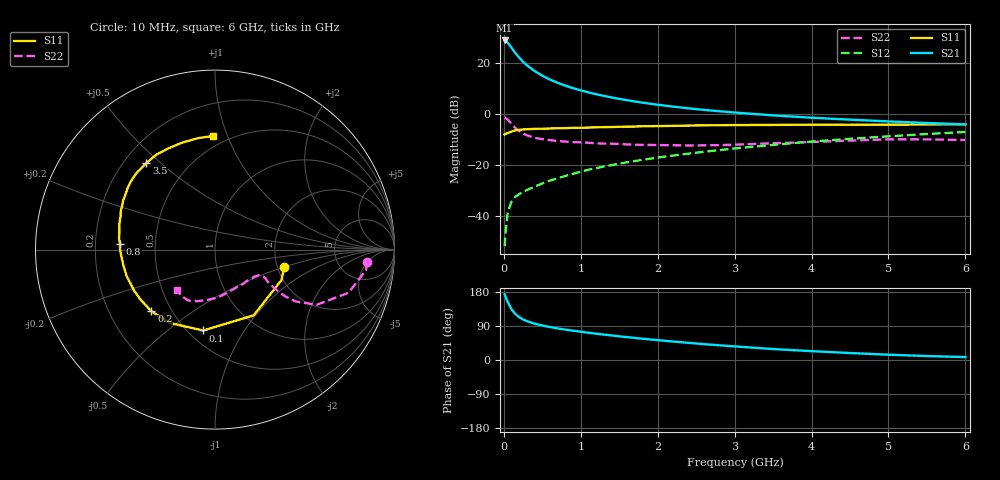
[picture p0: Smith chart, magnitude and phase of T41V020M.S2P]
! Infineon Technologies  Discrete & RF Semiconductors
! BFR182T
! Si NPN RF Bipolar Junction Transistor in SC75
! VCE = 1 V  IC = 20 mA
! Common Emitter S-Parameters:  October  1999
# GHz  S  MA  R  50
!  f  S11  S21  S12  S22
! GHz  MAG  ANG  MAG  ANG  MAG  ANG  MAG  ANG
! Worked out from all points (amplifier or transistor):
!   36 points, 10 MHz to 6 GHz, reference 50 ohm
!   highest |S21| = 29.1 dB at 10 MHz (marker M1)
!   |S21| within 3 dB of that: start of sweep to 102.8 MHz
!   unconditionally stable (mu >= 1): start of sweep to 18.1 MHz; 280.5 MHz to end of sweep
!   at 250 MHz: K = 0.94, MSG = 25.7 dB, |S12| = -30.7 dB
!   at 1.4 GHz: K = 1.48, MAG = 9.3 dB, |S12| = -20.1 dB
!   at 6 GHz: K = 1.11, MAG = -0.5 dB, |S12| = -7.0 dB
!   S11 on the Smith chart (normalised r, x): 10 MHz: 2.18, -0.50; 100 MHz: 0.59, -0.67; 200 MHz: 0.39, -0.35; 800 MHz: 0.31, +0.03; 3.5 GHz: 0.29, +0.45; 6 GHz: 0.42, +0.89
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0.01  0.398 -14.2  28.47 173.3  0.0025 79.6  0.8494 -4.6
0.02  0.4075 -24.6  28.24 168.7  0.0043 88.5  0.8492 -7.7
0.05  0.4251 -59.5  25.81 152.9  0.0114 73.6  0.7822 -17.9
0.1  0.4554 -98.3  20.43 133.7  0.019 60.3  0.6445 -28.5
0.15  0.4807 -121.8  16.07 121.1  0.0237 55.7  0.5353 -32.7
0.2  0.4932 -135.9  13.01 112.9  0.0266 55.8  0.4648 -33.7
0.25  0.4998 -145.8  10.83 107.0  0.0292 54.3  0.4152 -33.3
0.3  0.5056 -153.2  9.224 102.5  0.032 55.3  0.3845 -32.8
0.4  0.5141 -163.3  7.099 95.8  0.0372 57.4  0.3419 -31.2
0.5  0.5178 -170.1  5.749 91.0  0.0431 61.1  0.3225 -29.6
0.6  0.5224 -175.3  4.811 86.9  0.049 62.6  0.3081 -29.2
0.7  0.5285 -179.6  4.159 83.4  0.0547 64.7  0.2963 -29.2
0.8  0.5306 176.5  3.659 80.1  0.0607 65.5  0.2882 -29.8
0.9  0.5389 173.2  3.26 77.4  0.0667 67.4  0.2817 -30.4
1.1  0.5457 167.4  2.694 71.9  0.0806 68.2  0.2733 -32.8
1.3  0.5555 162.5  2.302 67.0  0.0933 69.0  0.2635 -35.9
1.6  0.5698 156.2  1.887 60.4  0.1127 69.1  0.2538 -41.3
2.2  0.5894 146.9  1.411 48.7  0.1533 68.5  0.2447 -55.5
3.5  0.6152 128.4  0.948 28.9  0.2486 62.5  0.2674 -86.9
4.5  0.6211 114.8  0.782 18.4  0.3277 55.3  0.3021 -108.2
5.5  0.6281 98.7  0.671 10.4  0.4068 46.8  0.3191 -125.3
6  0.6333 90.8  0.63 7.7  0.4461 41.7  0.3098 -133.5
